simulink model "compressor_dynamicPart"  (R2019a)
settings: Solver=VariableStepAuto  StartTime=0.0  StopTime=tend  RelTol=1e-3
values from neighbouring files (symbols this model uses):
  mc = 9.7005    [Compressor_dynamicPart_test.m]    (also in compressor.m = Qc*rho_a)
  omega0 = 13370    [Compressor_dynamicPart_test.m]
  p = [kt_Rm, eta_motor, kappa_v, eta_c, J_c, cp_a, kappa_a, T_amb]    [Compressor_dynamicPart_test.m]
  P_ratio = 2.1    [Compressor_dynamicPart_test.m]    (also in flow2omega.m = u(2); compressor.m = u(2))
  Tstep1 = 10    [Compressor_dynamicPart_test.m]
  V0 = 170    [Compressor_dynamicPart_test.m]    (also in colamod.m = 3.20629; ColumnA_simulation.m = 3.20629)
  Vstep1 = V0*0    (= 0)    [Compressor_dynamicPart_test.m]
undefined symbols (not defined in the file or in its folder): compressor_motor, tipspeed

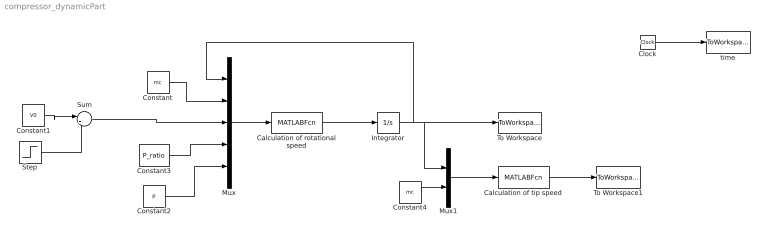
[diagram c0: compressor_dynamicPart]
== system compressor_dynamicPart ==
  Calculation of rotational speed : MATLABFcn  MATLABFcn=compressor_motor(u(1),u(2),u(3),u(4),u(5:12))  OutputDimensions=1
  Calculation of tip speed : MATLABFcn  MATLABFcn=tipspeed(u(1),u(2))  OutputDimensions=1
  Clock : Clock
  Constant : Constant  Value=mc
  Constant1 : Constant  Value=V0
  Constant2 : Constant  Value=p
  Constant3 : Constant  Value=P_ratio
  Constant4 : Constant  Value=mc
  Integrator : Integrator  InitialCondition=omega0
  Mux : Mux  Inputs=5
  Mux1 : Mux  Inputs=2
  Step : Step  Time=Tstep1  After=Vstep1  SampleTime=0
  Sum : Sum  Inputs=|++
  To Workspace : ToWorkspace  VariableName=omega  SampleTime=-1
  To Workspace1 : ToWorkspace  VariableName=Uc_out  SampleTime=-1
  time : ToWorkspace  VariableName=t  SampleTime=-1
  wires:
  Clock/1 -> time/1
  Constant/1 -> Mux/2
  Mux/1 -> Calculation of rotational speed/1
  Calculation of rotational speed/1 -> Integrator/1
  Integrator/1 -> Mux1/1, To Workspace/1, Mux/1
  Constant2/1 -> Mux/5
  Constant3/1 -> Mux/4
  Calculation of tip speed/1 -> To Workspace1/1
  Mux1/1 -> Calculation of tip speed/1
  Constant4/1 -> Mux1/2
  Step/1 -> Sum/2
  Constant1/1 -> Sum/1
  Sum/1 -> Mux/3
